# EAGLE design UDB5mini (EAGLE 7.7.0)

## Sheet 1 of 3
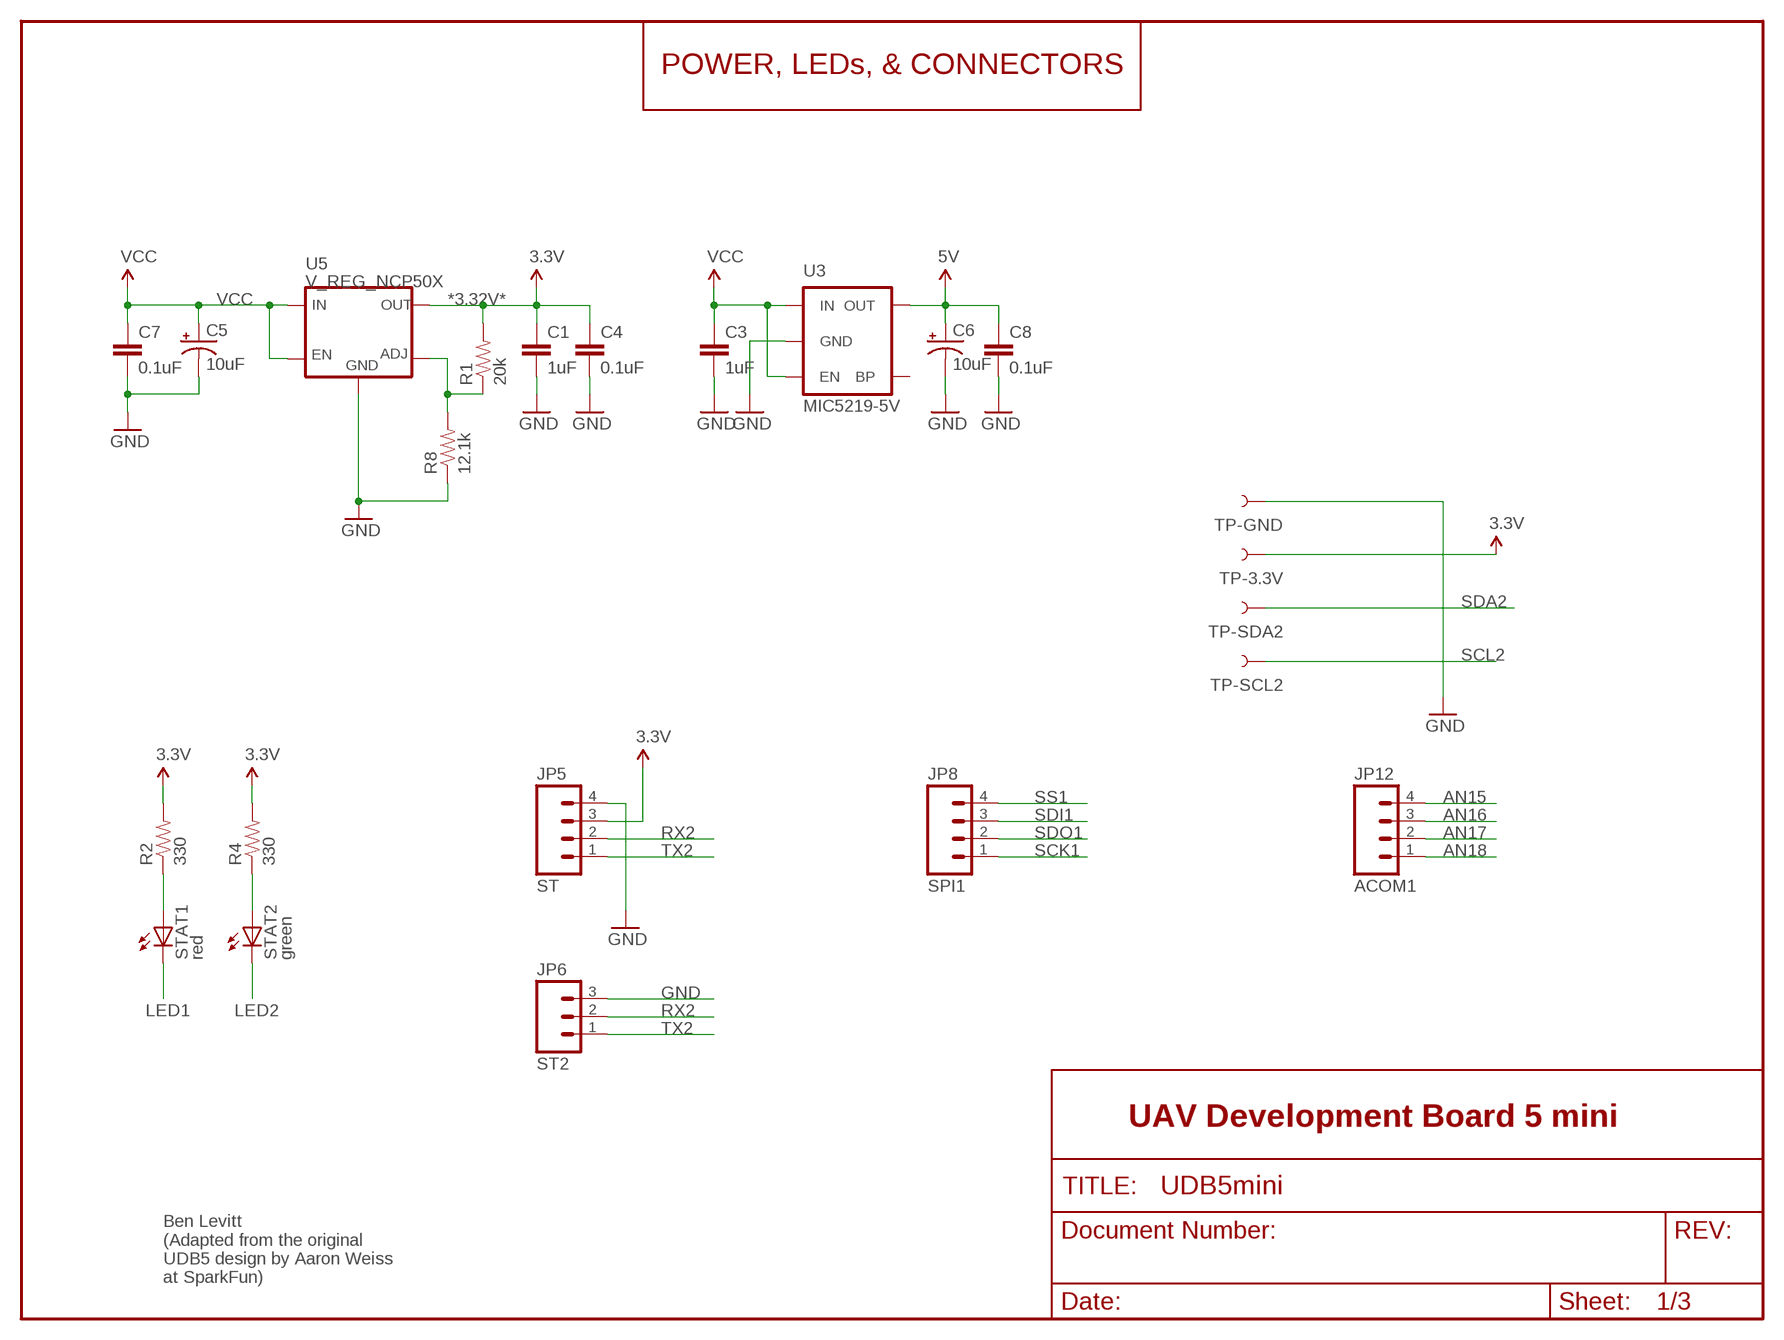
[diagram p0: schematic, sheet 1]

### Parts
C1  1uF  CAP0402-CAP  [0402-CAP]
C3  1uF  CAP0402-CAP  [0402-CAP]
C4  0.1uF  CAP0402-CAP  [0402-CAP]
C5  10uF  CAP_POL1206  [EIA3216]
C6  10uF  CAP_POL1206  [EIA3216]
C7  0.1uF  CAP0402-CAP  [0402-CAP]
C8  0.1uF  CAP0402-CAP  [0402-CAP]
JP5  ST  M04PTH  [1X04]
JP6  ST2  M03PTH  [1X03]
JP8  SPI1  M04PTH  [1X04]
JP12  ACOM1  M04PTH  [1X04]
R1  20k  RESISTOR0402-RES  [0402-RES]
R2  330  RESISTOR0402-RES  [0402-RES]
R4  330  RESISTOR0402-RES  [0402-RES]
R8  12.1k  RESISTOR0402-RES  [0402-RES]
STAT1  red  LED0603  [LED-0603]
STAT2  green  LED0603  [LED-0603]
TP-3.3V  TEST-POINT3X5  [PAD.03X.05]
TP-GND  TEST-POINT3X5  [PAD.03X.05]
TP-SCL2  TEST-POINT3X5  [PAD.03X.05]
TP-SDA2  TEST-POINT3X5  [PAD.03X.05]
U3  V_REG_LDOSMD  [SOT23-5]
U5  V_REG_NCP50X  [DPAK-5]

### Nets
3.3V: C1.1 C4.1 JP5.3 R1.2 R2.2 R4.2 TP-3.3V.P$1 U5.VOUT(OUT) ; also sheet 2,3
5V: C6.A(+) C8.1 U3.5(OUT) ; also sheet 3
AN15: JP12.4 ; also sheet 2
AN16: JP12.3 ; also sheet 2
AN17: JP12.2 ; also sheet 2
AN18: JP12.1 ; also sheet 2
GND: C1.2 C3.2 C4.2 C5.C(-) C6.C(-) C7.2 C8.2 JP5.4 JP6.3 R8.1 TP-GND.P$1 U3.2(GND) U5.GND ; also sheet 2,3
LED1: STAT1.C ; also sheet 2
LED2: STAT2.C ; also sheet 2
N$1: R2.1 STAT1.A
N$2: R4.1 STAT2.A
N$9: R1.1 R8.2 U5.ADJ
RX2: JP5.2 JP6.2 ; also sheet 2
SCK1: JP8.1 ; also sheet 2
SCL2: TP-SCL2.P$1 ; also sheet 2
SDA2: TP-SDA2.P$1 ; also sheet 2
SDI1: JP8.3 ; also sheet 2
SDO1: JP8.2 ; also sheet 2
SS1: JP8.4 ; also sheet 2
TX2: JP5.1 JP6.1 ; also sheet 2
VCC: C3.1 C5.A(+) C7.1 U3.1(IN) U3.4(EN) U5.EN U5.VIN(IN) ; also sheet 3
Unconnected: U3.3(BP)

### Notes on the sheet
- POWER, LEDs, & CONNECTORS
- *3.32V*
- MIC5219-5V
- UAV Development Board 5 mini
- Ben Levitt
  (Adapted from the original
  UDB5 design by Aaron Weiss
  at SparkFun)

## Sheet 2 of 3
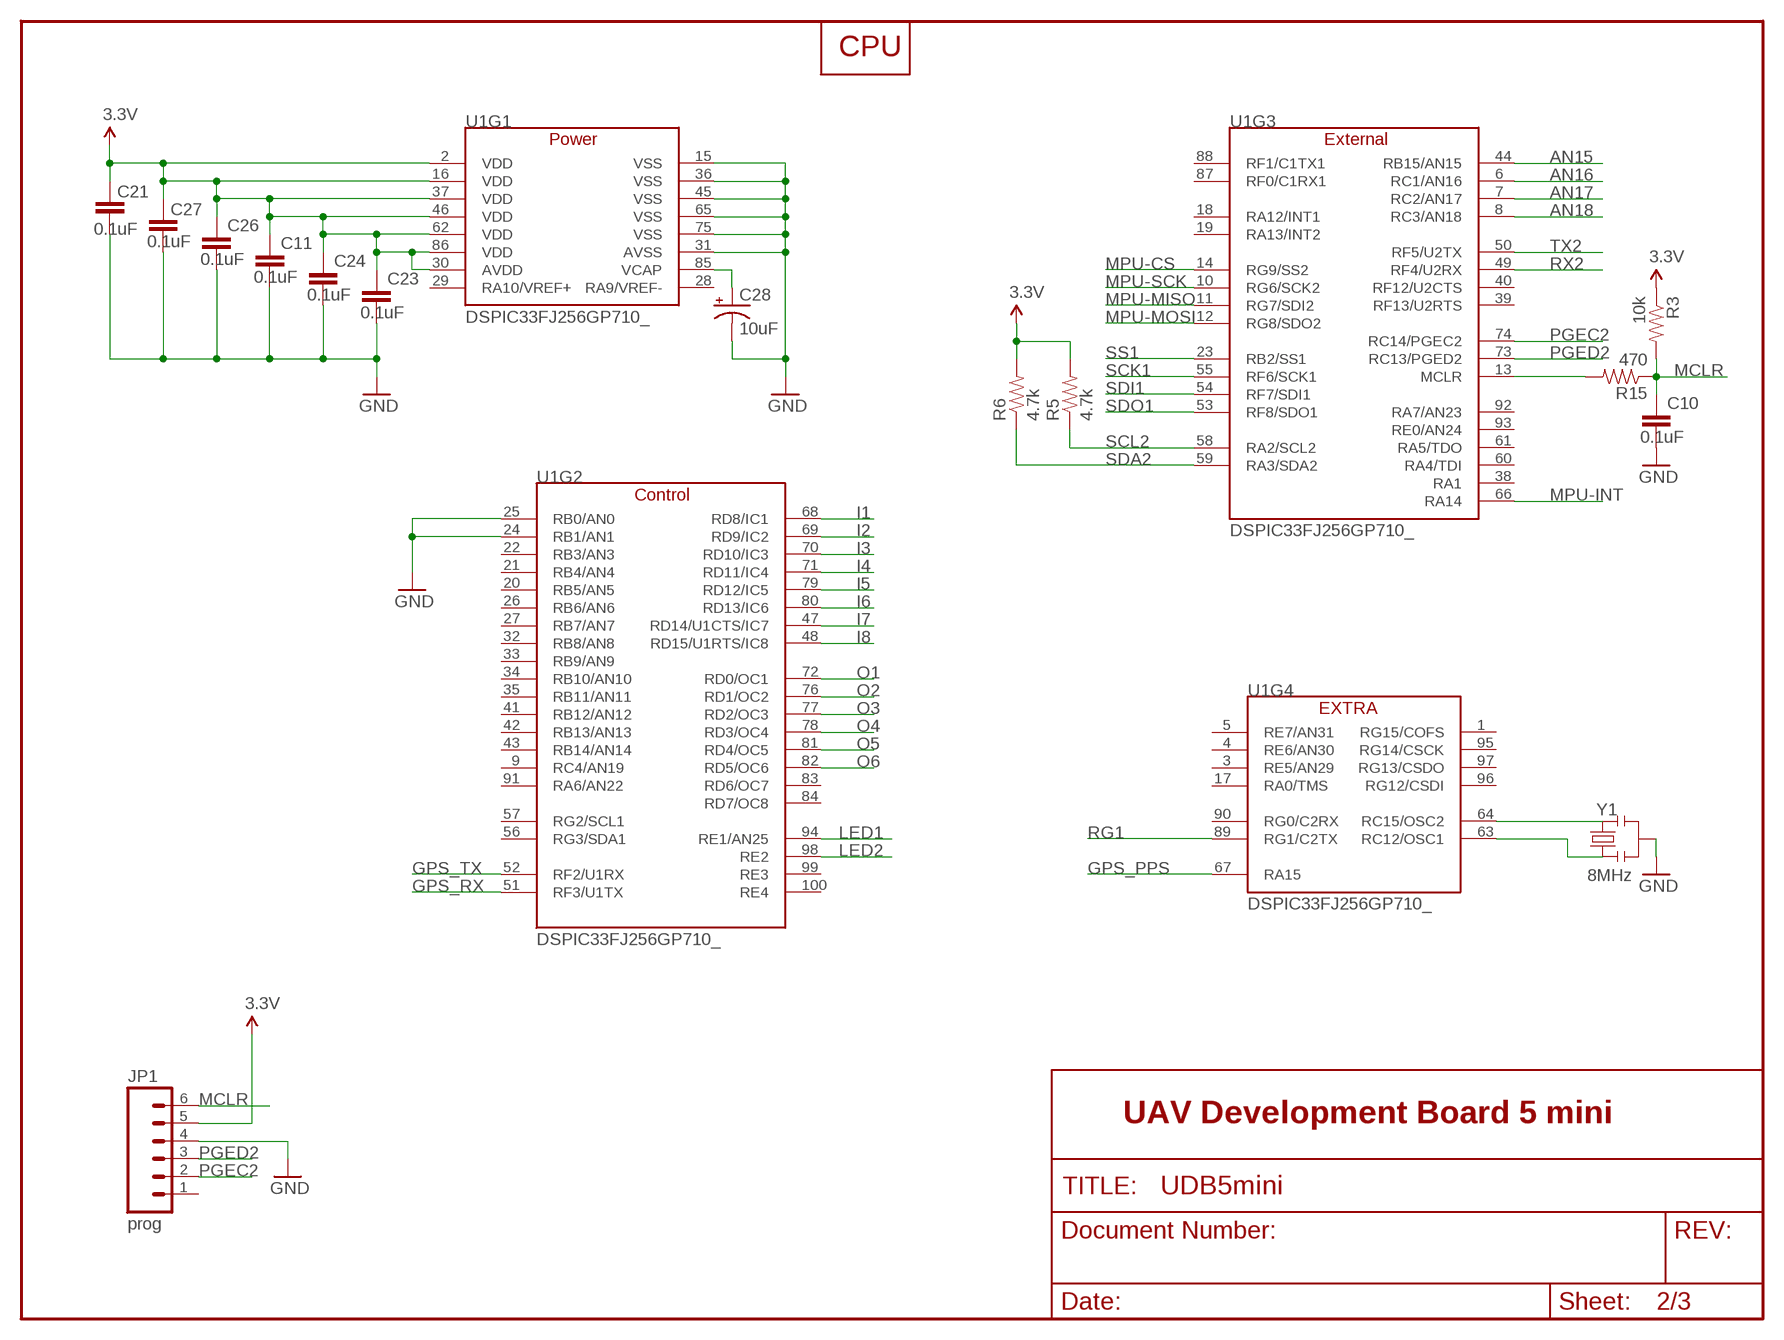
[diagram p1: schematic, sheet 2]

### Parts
C10  0.1uF  CAP0402-CAP  [0402-CAP]
C11  0.1uF  CAP0402-CAP  [0402-CAP]
C21  0.1uF  CAP0402-CAP  [0402-CAP]
C23  0.1uF  CAP0402-CAP  [0402-CAP]
C24  0.1uF  CAP0402-CAP  [0402-CAP]
C26  0.1uF  CAP0402-CAP  [0402-CAP]
C27  0.1uF  CAP0402-CAP  [0402-CAP]
C28  10uF  CAP_POL1206  [EIA3216]
JP1  prog  M06SIP  [1X06]
R3  10k  RESISTOR0402-RES  [0402-RES]
R5  4.7k  RESISTOR0402-RES  [0402-RES]
R6  4.7k  RESISTOR0402-RES  [0402-RES]
R15  470  RESISTOR0402-RES  [0402-RES]
U1  DSPIC33FJ256GP710_  [TQFP-100-12X12MM]
Y1  RESONATORSMD  [RESONATOR-SMD]

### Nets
3.3V: C11.1 C21.1 C23.1 C24.1 C26.1 C27.1 JP1.5 R3.1 R5.2 R6.2 U1.2(VDD) U1.16(VDD) U1.30(AVDD) U1.37(VDD) U1.46(VDD) U1.62(VDD) U1.86(VDD) ; also sheet 1,3
AN15: U1.44(RB15/AN15) ; also sheet 1
AN16: U1.6(RC1/AN16) ; also sheet 1
AN17: U1.7(RC2/AN17) ; also sheet 1
AN18: U1.8(RC3/AN18) ; also sheet 1
GND: C10.2 C11.2 C21.2 C23.2 C24.2 C26.2 C27.2 C28.C(-) JP1.4 U1.15(VSS) U1.24(RB1/AN1) U1.25(RB0/AN0) U1.31(AVSS) U1.36(VSS) U1.45(VSS) U1.65(VSS) U1.75(VSS) Y1.2 ; also sheet 1,3
GPS_PPS: U1.67(RA15) ; also sheet 3
GPS_RX: U1.51(RF3/U1TX) ; also sheet 3
GPS_TX: U1.52(RF2/U1RX) ; also sheet 3
I1: U1.68(RD8/IC1) ; also sheet 3
I2: U1.69(RD9/IC2) ; also sheet 3
I3: U1.70(RD10/IC3) ; also sheet 3
I4: U1.71(RD11/IC4) ; also sheet 3
I5: U1.79(RD12/IC5) ; also sheet 3
I6: U1.80(RD13/IC6) ; also sheet 3
I7: U1.47(RD14/U1CTS/IC7) ; also sheet 3
I8: U1.48(RD15/U1RTS/IC8) ; also sheet 3
LED1: U1.94(RE1/AN25) ; also sheet 1
LED2: U1.98(RE2) ; also sheet 1
MCLR: C10.1 JP1.6 R3.2 R15.1
MPU-CS: U1.14(RG9/SS2) ; also sheet 3
MPU-INT: U1.66(RA14) ; also sheet 3
MPU-MISO: U1.11(RG7/SDI2) ; also sheet 3
MPU-MOSI: U1.12(RG8/SDO2) ; also sheet 3
MPU-SCK: U1.10(RG6/SCK2) ; also sheet 3
N$3: U1.64(RC15/OSC2) Y1.3
N$6: U1.63(RC12/OSC1) Y1.1
N$7: R15.2 U1.13(MCLR)
N$35: C28.A(+) U1.85(VCAP)
O1: U1.72(RD0/OC1) ; also sheet 3
O2: U1.76(RD1/OC2) ; also sheet 3
O3: U1.77(RD2/OC3) ; also sheet 3
O4: U1.78(RD3/OC4) ; also sheet 3
O5: U1.81(RD4/OC5) ; also sheet 3
O6: U1.82(RD5/OC6) ; also sheet 3
PGEC2: JP1.2 U1.74(RC14/PGEC2)
PGED2: JP1.3 U1.73(RC13/PGED2)
RG1: U1.89(RG1/C2TX) ; also sheet 3
RX2: U1.49(RF4/U2RX) ; also sheet 1
SCK1: U1.55(RF6/SCK1) ; also sheet 1
SCL2: R5.1 U1.58(RA2/SCL2) ; also sheet 1
SDA2: R6.1 U1.59(RA3/SDA2) ; also sheet 1
SDI1: U1.54(RF7/SDI1) ; also sheet 1
SDO1: U1.53(RF8/SDO1) ; also sheet 1
SS1: U1.23(RB2/SS1) ; also sheet 1
TX2: U1.50(RF5/U2TX) ; also sheet 1
Unconnected: JP1.1 U1.1(RG15/COFS) U1.3(RE5/AN29) U1.4(RE6/AN30) U1.5(RE7/AN31) U1.9(RC4/AN19) U1.17(RA0/TMS) U1.18(RA12/INT1) U1.19(RA13/INT2) U1.20(RB5/AN5) U1.21(RB4/AN4) U1.22(RB3/AN3) U1.26(RB6/AN6) U1.27(RB7/AN7) U1.28(RA9/VREF-) U1.29(RA10/VREF+) U1.32(RB8/AN8) U1.33(RB9/AN9) U1.34(RB10/AN10) U1.35(RB11/AN11) U1.38(RA1) U1.39(RF13/U2RTS) U1.40(RF12/U2CTS) U1.41(RB12/AN12) U1.42(RB13/AN13) U1.43(RB14/AN14) U1.56(RG3/SDA1) U1.57(RG2/SCL1) U1.60(RA4/TDI) U1.61(RA5/TDO) U1.83(RD6/OC7) U1.84(RD7/OC8) U1.87(RF0/C1RX1) U1.88(RF1/C1TX1) U1.90(RG0/C2RX) U1.91(RA6/AN22) U1.92(RA7/AN23) U1.93(RE0/AN24) U1.95(RG14/CSCK) U1.96(RG12/CSDI) U1.97(RG13/CSDO) U1.99(RE3) U1.100(RE4)

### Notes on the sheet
- CPU
- 8MHz
- UAV Development Board 5 mini

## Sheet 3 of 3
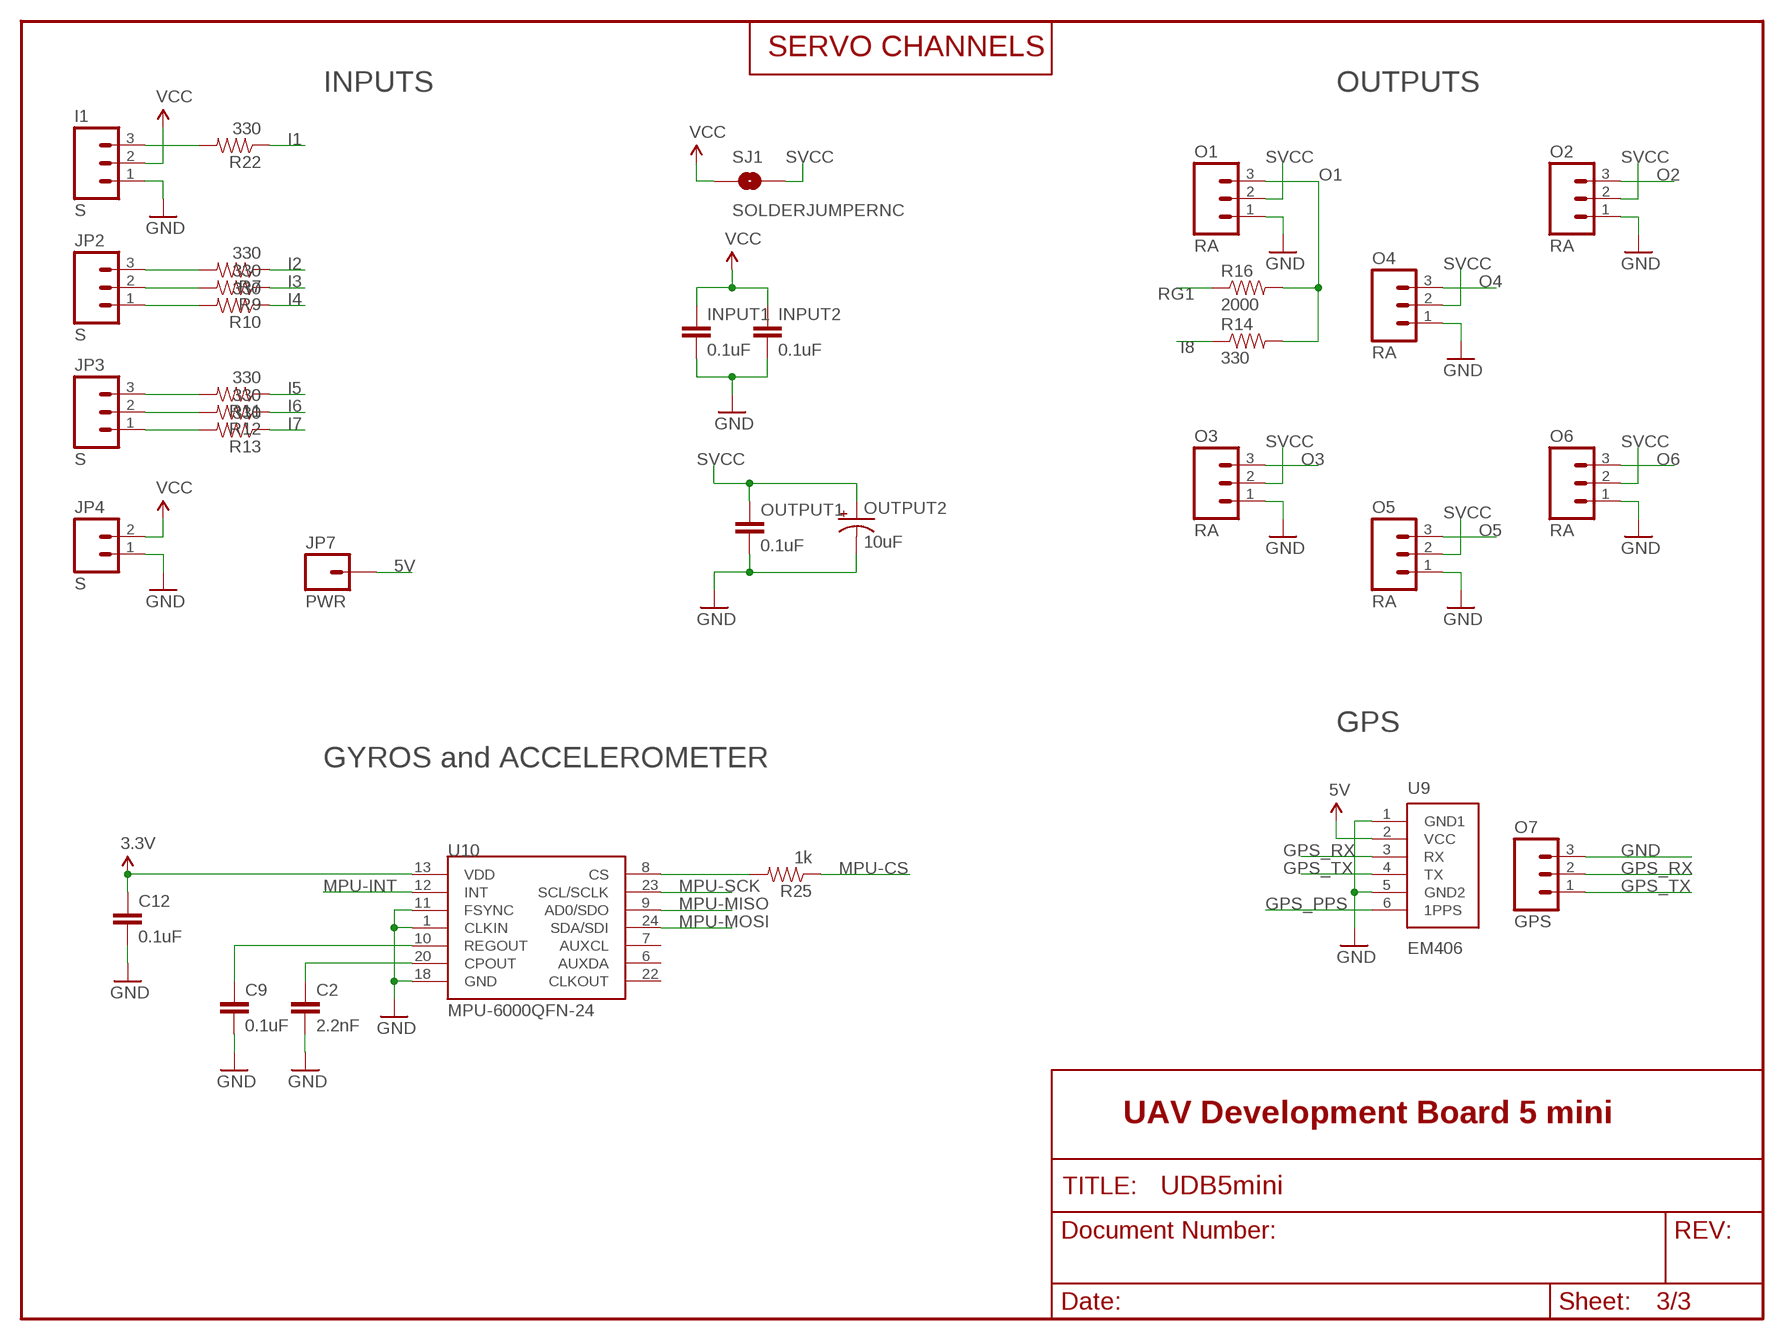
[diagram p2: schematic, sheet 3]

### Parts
C2  2.2nF  CAP0402-CAP  [0402-CAP]
C9  0.1uF  CAP0402-CAP  [0402-CAP]
C12  0.1uF  CAP0402-CAP  [0402-CAP]
I1  S  M03PTH  [1X03]
INPUT1  0.1uF  CAP0402-CAP  [0402-CAP]
INPUT2  0.1uF  CAP0402-CAP  [0402-CAP]
JP2  S  M03PTH  [1X03]
JP3  S  M03PTH  [1X03]
JP4  S  M02PTH  [1X02]
JP7  PWR  M01PTH  [1X01]
O1  RA  M03PTH  [1X03]
O2  RA  M03PTH  [1X03]
O3  RA  M03PTH  [1X03]
O4  RA  M03PTH  [1X03]
O5  RA  M03PTH  [1X03]
O6  RA  M03PTH  [1X03]
O7  GPS  M03PTH  [1X03]
OUTPUT1  0.1uF  CAP0402-CAP  [0402-CAP]
OUTPUT2  10uF  CAP_POL1206  [EIA3216]
R7  330  RESISTOR0402-RES  [0402-RES]
R9  330  RESISTOR0402-RES  [0402-RES]
R10  330  RESISTOR0402-RES  [0402-RES]
R11  330  RESISTOR0402-RES  [0402-RES]
R12  330  RESISTOR0402-RES  [0402-RES]
R13  330  RESISTOR0402-RES  [0402-RES]
R14  330  RESISTOR0402-RES  [0402-RES]
R16  2000  RESISTOR0402-RES  [0402-RES]
R22  330  RESISTOR0402-RES  [0402-RES]
R25  1k  RESISTOR0402-RES  [0402-RES]
SJ1  SOLDERJUMPERNC  [SJ_2S]
U9  EM406  [EM406]
U10  MPU-6000QFN-24  [QFN-24-TESTING]

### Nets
3.3V: C12.1 U10.13(VDD) ; also sheet 1,2
5V: JP7.1 U9.2(VCC) ; also sheet 1
GND: C2.2 C9.2 C12.2 I1.1 INPUT1.2 INPUT2.2 JP4.1 O1.1 O2.1 O3.1 O4.1 O5.1 O6.1 O7.3 OUTPUT1.2 OUTPUT2.C(-) U9.1(GND1) U9.5(GND2) U10.1(CLKIN) U10.11(FSYNC) U10.18(GND) ; also sheet 1,2
GPS_PPS: U9.6(1PPS) ; also sheet 2
GPS_RX: O7.2 U9.3(RX) ; also sheet 2
GPS_TX: O7.1 U9.4(TX) ; also sheet 2
I1: R22.1 ; also sheet 2
I2: R7.1 ; also sheet 2
I3: R9.1 ; also sheet 2
I4: R10.1 ; also sheet 2
I5: R11.1 ; also sheet 2
I6: R12.1 ; also sheet 2
I7: R13.1 ; also sheet 2
I8: R14.1 ; also sheet 2
MPU-CS: R25.1 ; also sheet 2
MPU-INT: U10.12(INT) ; also sheet 2
MPU-MISO: U10.9(AD0/SDO) ; also sheet 2
MPU-MOSI: U10.24(SDA/SDI) ; also sheet 2
MPU-SCK: U10.23(SCL/SCLK) ; also sheet 2
N$4: JP2.3 R7.2
N$5: R25.2 U10.8(CS)
N$8: JP2.2 R9.2
N$10: JP2.1 R10.2
N$11: JP3.3 R11.2
N$12: JP3.2 R12.2
N$13: C2.1 U10.20(CPOUT)
N$14: JP3.1 R13.2
N$16: C9.1 U10.10(REGOUT)
N$21: I1.3 R22.2
O1: O1.3 R14.2 R16.2 ; also sheet 2
O2: O2.3 ; also sheet 2
O3: O3.3 ; also sheet 2
O4: O4.3 ; also sheet 2
O5: O5.3 ; also sheet 2
O6: O6.3 ; also sheet 2
RG1: R16.1 ; also sheet 2
SVCC: O1.2 O2.2 O3.2 O4.2 O5.2 O6.2 OUTPUT1.1 OUTPUT2.A(+) SJ1.2
VCC: I1.2 INPUT1.1 INPUT2.1 JP4.2 SJ1.1 ; also sheet 1
Unconnected: U10.6(AUXDA) U10.7(AUXCL) U10.22(CLKOUT)

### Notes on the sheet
- SERVO CHANNELS
- INPUTS | OUTPUTS
- GPS
- GYROS and ACCELEROMETER
- UAV Development Board 5 mini

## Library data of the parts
C1 C3 C4 C7 C8 C10 C11 C21 C23 C24 C26 C27 INPUT1 INPUT2 OUTPUT1 = SparkFun:CAP: Capacitor
C2 C9 C12 = SparkFun-Capacitors:CAP: Capacitor
C5 C6 C28 OUTPUT2 = SparkFun:CAP_POL: Capacitor Polarized
I1 JP2 JP3 O1-O7 = SparkFun:M03: Header 3 Standard 3-pin 0.1" header. Use with straight break away headers (SKU : PRT-00116), right angle break away headers (PRT-00553), swiss pins (PRT-00743), machine pins (PRT-00117), and female headers (PRT-00115). Molex polarized connector foot print use with SKU : PRT-08232 with associated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
JP1 = SparkFun:M06: Header 6 Standard 6-pin 0.1" header. Use with straight break away headers (SKU : PRT-00116), right angle break away headers (PRT-00553), swiss pins (PRT-00743), machine pins (PRT-00117), and female headers (PRT-00115). Molex polarized connector foot print use with SKU : PRT-08094 with associated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
JP4 = SparkFun-Connectors:M02: Standard 2-pin 0.1" header. Use with
JP5 JP8 JP12 = udb5mini:M04: Header 4 Standard 4-pin 0.1" header. Use with straight break away headers (SKU : PRT-00116), right angle break away headers (PRT-00553), swiss pins (PRT-00743), machine pins (PRT-00117), and female headers (PRT-00115). Molex polarized connector foot print use with SKU : PRT-08231 with associated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
JP6 = SparkFun-Connectors:M03: Header 3 Standard 3-pin 0.1" header. Use with straight break away headers (SKU : PRT-00116), right angle break away headers (PRT-00553), swiss pins (PRT-00743), machine pins (PRT-00117), and female headers (PRT-00115). Molex polarized connector foot print use with SKU : PRT-08232 with associated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
JP7 = SparkFun-Connectors:M01: Header 1
R1-R16 R22 R25 = SparkFun:RESISTOR: Resistor
SJ1 = SparkFun:SOLDERJUMPER: Solder Jumper
STAT1 STAT2 = SparkFun:LED: LEDs
TP-3.3V TP-GND TP-SCL2 TP-SDA2 = SparkFun-Passives:TEST-POINT: Bare copper test points for troubleshooting or ICT
U1 = SparkFun:DSPIC33FJ256GP710
U3 = SparkFun-PowerIC:V_REG_LDO: Voltage Regulator LDO Standard 150mA LDO voltage regulator in SOT-23 layout. Micrel part MIC5205. BP (by-pass) pin is used to lower output noise with 470pF cap.
U5 = SparkFun:V_REG_NCP50X: NCP550x 500mA LDO Voltage Regulator
U9 = SparkFun:EM406: EM406 Connector Proven layout and schematic for EM406 connector. Spark Fun Electronics SKU : GPS-00579
U10 = SparkFun-Sensors:MPU-6000: MPU-6000 - I2C address is 0x68 with AD0 low and 0x69 with AD0 high.
Y1 = SparkFun:RESONATOR: Resonator Small SMD resonator. This is the itty bitty 10/20MHz resonators with built in caps. CSTCE10M0G55 and CSTCE20M0V53. Footprint has been reviewed closely but hasn't been tested yet.

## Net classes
1 antenna: width 2.974 mm

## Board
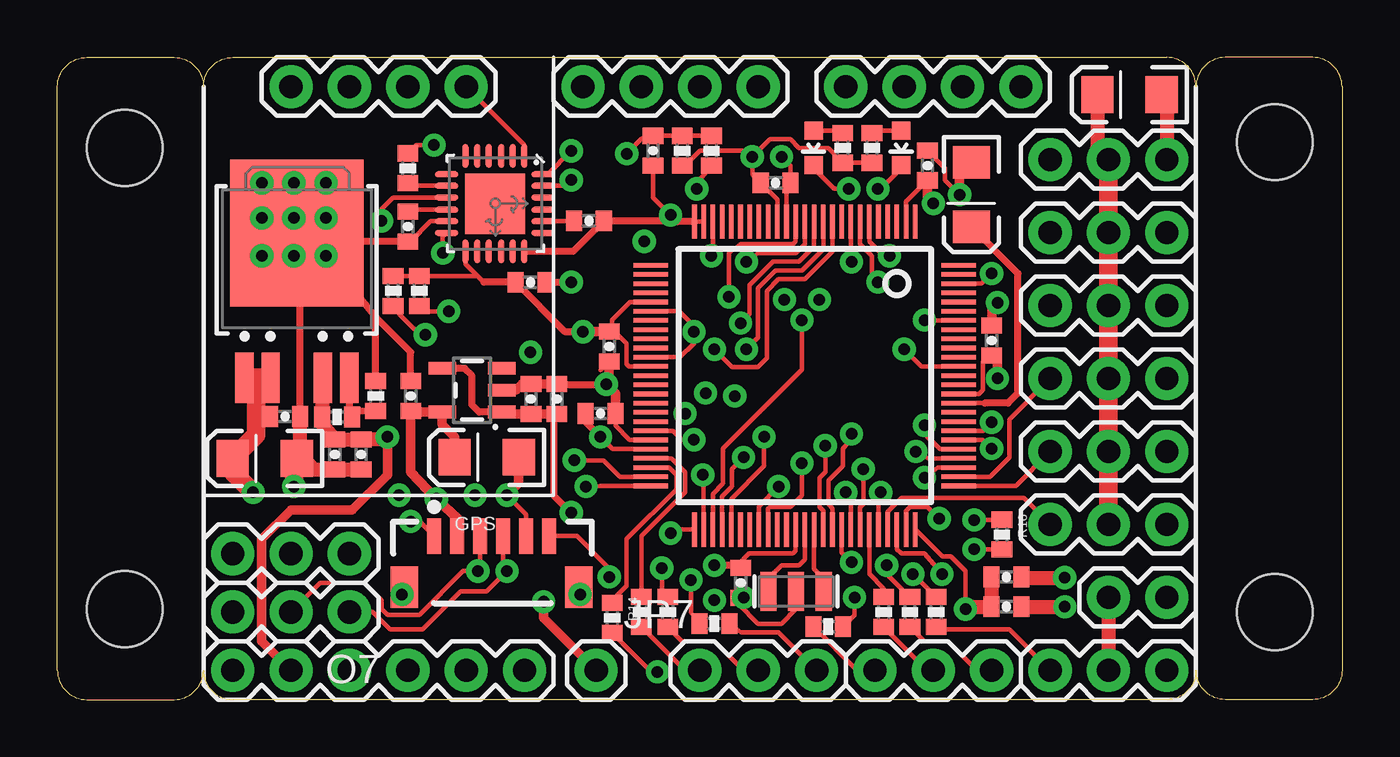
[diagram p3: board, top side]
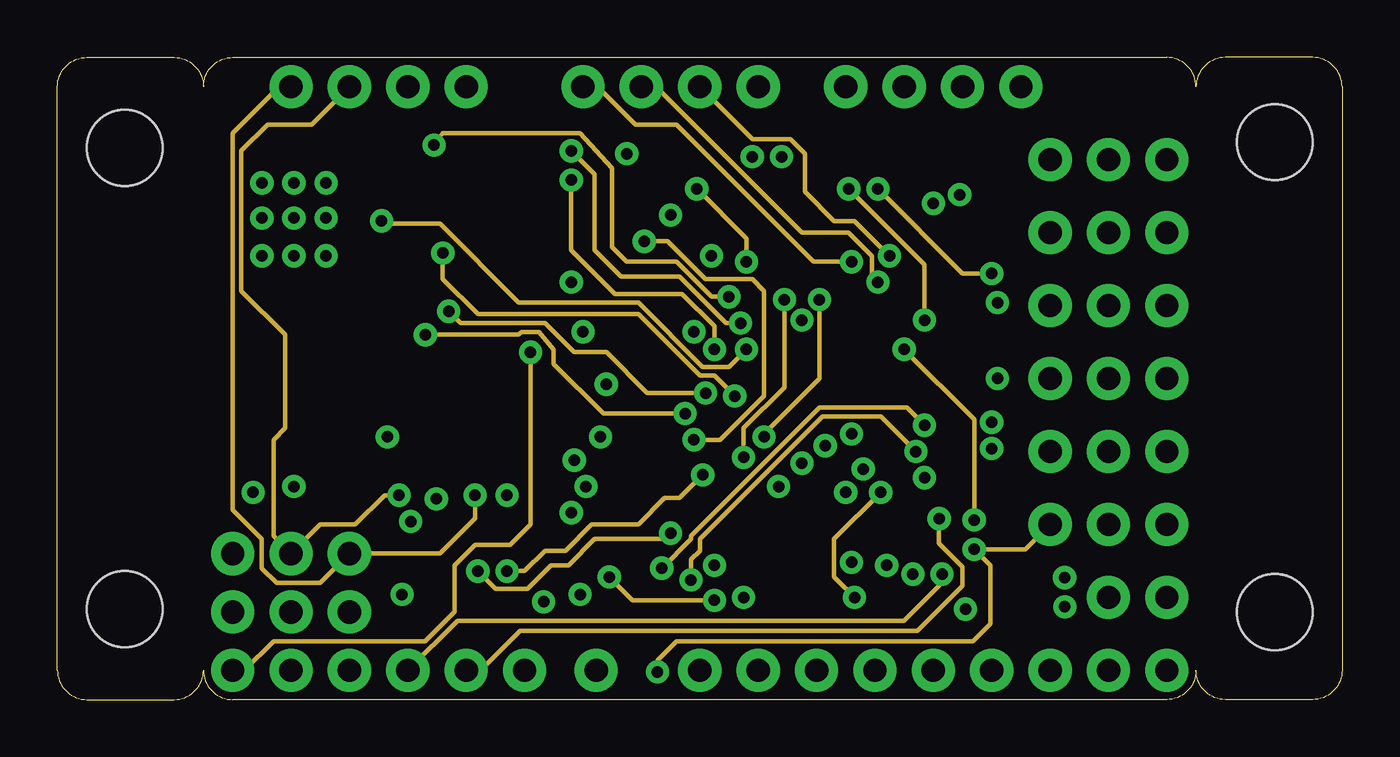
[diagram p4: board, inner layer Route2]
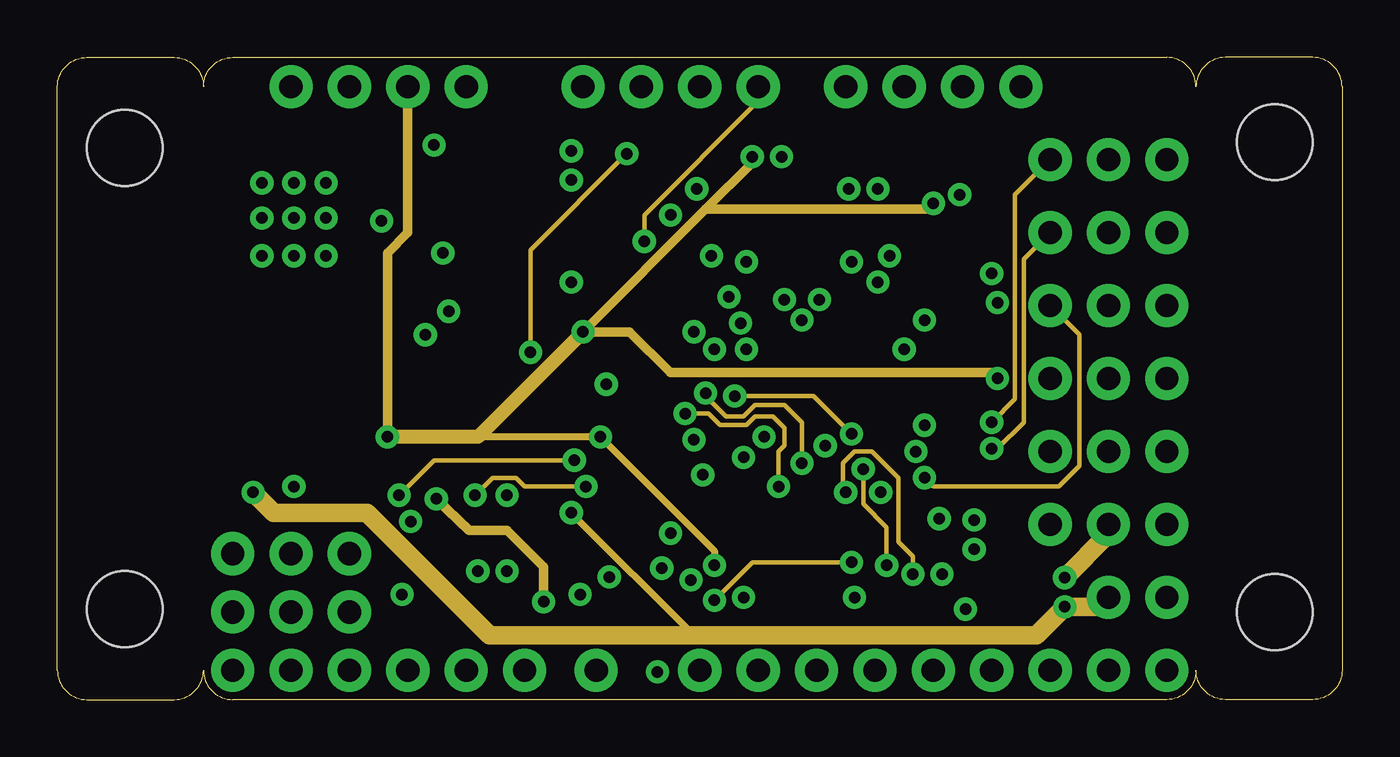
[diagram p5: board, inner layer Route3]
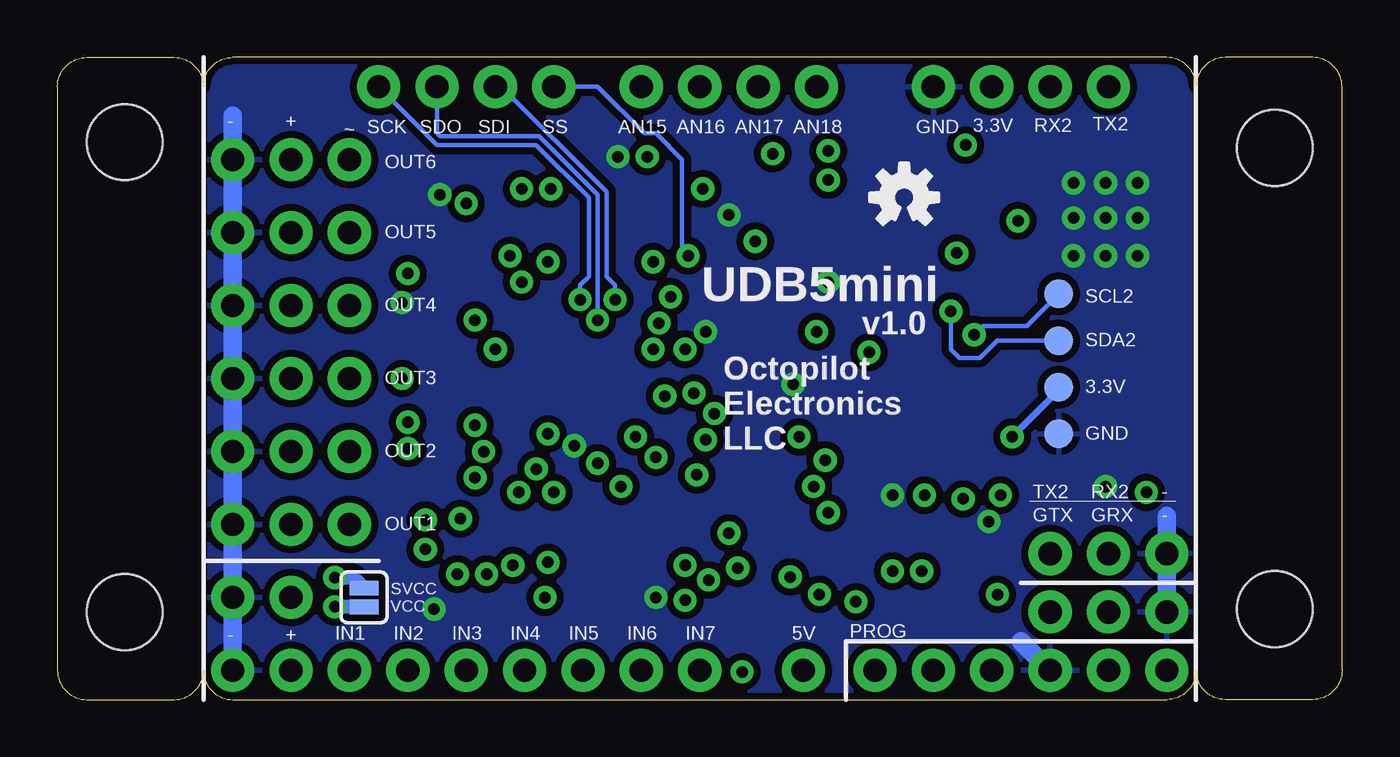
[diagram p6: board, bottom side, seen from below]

Size 55.88 x 27.94 mm. Coordinates in mm from the lower left corner, seen from the top.
Outline: 0,1.27 0,26.67 arc-90 1.27,27.94 5.08,27.94 arc-90 6.35,26.67 arc-90 7.62,27.94 48.26,27.94 arc-90 49.53,26.67 arc-90 50.8,27.94 54.61,27.94 arc-90 55.88,26.67 55.88,1.27 arc-90 54.61,0 50.8,0 arc-90 49.53,1.27 arc-90 48.26,0 7.62,0 arc-90 6.35,1.27 arc-90 5.08,0 1.27,0 arc-90 0,1.27
Copper layers (1*2*3*16): Top 0.035mm / dielectric 0.23mm / Route2 0.035mm / dielectric 0.93mm / Route3 0.035mm / dielectric 0.23mm / Bottom 0.035mm
Design rules "BatchPCB-4-layer *": minimum track width 5mil, minimum drill 12mil, track to track 5mil, track to pad 5mil, pad to pad 5mil, via to via 5mil, smd to smd 5mil, copper to edge 8mil, drill to drill 12mil, minimum pad ring 12mil, minimum via ring 10mil, stop-mask expansion 4mil, vias tented up to drill 20mil, thermal gap 12mil

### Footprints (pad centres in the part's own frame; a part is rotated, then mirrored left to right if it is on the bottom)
0402-CAP = smd 0.7 x 0.9: 1 -0.65,0; 2 0.65,0
EIA3216 = smd 1.4 x 1.6: A 1.4,0; C -1.4,0
1X03 = drill 1.016 pad 1.88: 1 0,0; 2 2.54,0; 3 5.08,0
1X06 = drill 1.016 pad 1.88: 1 0,0; 2 2.54,0; 3 5.08,0; 4 7.62,0; 5 10.16,0; 6 12.7,0
1X02 = drill 1.016 pad 1.88: 1 0,0; 2 2.54,0
1X04 = drill 1.016 pad 1.88: 1 0,0; 2 2.54,0; 3 5.08,0; 4 7.62,0
1X01 = drill 1.016 pad 1.88: 1 0,0
0402-RES = smd 0.7 x 0.9: 1 -0.65,0; 2 0.65,0
SJ_2S = smd 0.635 x 1.27: 1 -0.412,0; 2 0.412,0
LED-0603 = smd 0.8 x 0.8: A 0,-0.75; C 0,0.75
PAD.03X.05 = smd 1.27 x 1.27: P$1 0,0
TQFP-100-12X12MM = smd 1.5 x 0.2: 1 -6.7,4.8; 2 -6.7,4.4; 3 -6.7,4; 4 -6.7,3.6; 5 -6.7,3.2; 6 -6.7,2.8; 7 -6.7,2.4; 8 -6.7,2; 9 -6.7,1.6; 10 -6.7,1.2; 11 -6.7,0.8; 12 -6.7,0.4; 13 -6.7,0; 14 -6.7,-0.4; 15 -6.7,-0.8; 16 -6.7,-1.2; 17 -6.7,-1.6; 18 -6.7,-2; 19 -6.7,-2.4; 20 -6.7,-2.8; 21 -6.7,-3.2; 22 -6.7,-3.6; 23 -6.7,-4; 24 -6.7,-4.4; 25 -6.7,-4.8; 51 6.7,-4.8; 52 6.7,-4.4; 53 6.7,-4; 54 6.7,-3.6; 55 6.7,-3.2; 56 6.7,-2.8; 57 6.7,-2.4; 58 6.7,-2; 59 6.7,-1.6; 60 6.7,-1.2; 61 6.7,-0.8; 62 6.7,-0.4; 63 6.7,0; 64 6.7,0.4; 65 6.7,0.8; 66 6.7,1.2; 67 6.7,1.6; 68 6.7,2; 69 6.7,2.4; 70 6.7,2.8; 71 6.7,3.2; 72 6.7,3.6; 73 6.7,4; 74 6.7,4.4; 75 6.7,4.8 | smd 0.2 x 1.5: 26 -4.8,-6.7; 27 -4.4,-6.7; 28 -4,-6.7; 29 -3.6,-6.7; 30 -3.2,-6.7; 31 -2.8,-6.7; 32 -2.4,-6.7; 33 -2,-6.7; 34 -1.6,-6.7; 35 -1.2,-6.7; 36 -0.8,-6.7; 37 -0.4,-6.7; 38 0,-6.7; 39 0.4,-6.7; 40 0.8,-6.7; 41 1.2,-6.7; 42 1.6,-6.7; 43 2,-6.7; 44 2.4,-6.7; 45 2.8,-6.7; 46 3.2,-6.7; 47 3.6,-6.7; 48 4,-6.7; 49 4.4,-6.7; 50 4.8,-6.7; 76 4.8,6.7; 77 4.4,6.7; 78 4,6.7; 79 3.6,6.7; 80 3.2,6.7; 81 2.8,6.7; 82 2.4,6.7; 83 2,6.7; 84 1.6,6.7; 85 1.2,6.7; 86 0.8,6.7; 87 0.4,6.7; 88 0,6.7; 89 -0.4,6.7; 90 -0.8,6.7; 91 -1.2,6.7; 92 -1.6,6.7; 93 -2,6.7; 94 -2.4,6.7; 95 -2.8,6.7; 96 -3.2,6.7; 97 -3.6,6.7; 98 -4,6.7; 99 -4.4,6.7; 100 -4.8,6.7
SOT23-5 = smd 0.55 x 1.2: 1 -0.95,-1.3; 2 0,-1.3; 3 0.95,-1.3; 4 0.95,1.3; 5 -0.95,1.3
DPAK-5 = smd 0.8 x 2.2: ADJ 2.28,-5.3; EN -2.28,-5.3; VIN -1.14,-5.3; VOUT 1.14,-5.3 | smd 5.8 x 6.4: GND 0,1
EM406 = smd 0.6 x 1.55: 1 0,0; 2 1,0; 3 2,0; 4 3,0; 5 4,0; 6 5,0 | smd 1.2 x 1.8: P$1 -1.3,-2.225; P$2 6.3,-2.225
QFN-24-TESTING = smd 1.016 x 0.254: 1 -2.066,1.257; 2 -2.066,0.75; 3 -2.066,0.247; 4 -2.066,-0.287; 5 -2.066,-0.792; 6 -2.066,-1.297; 13 2.086,-1.297; 14 2.086,-0.792; 15 2.086,-0.287; 16 2.086,0.247; 17 2.086,0.75; 18 2.086,1.257 | smd 0.254 x 1.016: 7 -1.267,-2.122; 8 -0.762,-2.122; 9 -0.258,-2.122; 10 0.278,-2.122; 11 0.78,-2.122; 12 1.287,-2.122; 19 1.287,2.082; 20 0.78,2.082; 21 0.278,2.082; 22 -0.258,2.082; 23 -0.762,2.082; 24 -1.267,2.082 | smd 2.616 x 2.616: P$1 0.02,-0.01
STAND-OFF = hole 3.302: 0,0
RESONATOR-SMD = smd 0.7 x 1.7: 1 -1.2,0; 2 0,0; 3 1.2,0

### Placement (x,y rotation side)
C1  12.06,10.67 270 top
C2  23.11,20.83 0 top
C3  21.72,13.08 90 top
C4  13.21,10.67 270 top
C5  9.02,10.49 180 top
C6  18.67,10.54 180 top
C7  9.91,12.32 0 top
C8  15.37,13.21 90 top
C9  15.24,20.57 270 top
C10  25.91,23.88 270 top
C11  23.62,12.45 0 top
C12  20.57,18.16 0 top
C21  37.85,23.24 90 top
C23  40.64,15.62 90 top
C24  29.72,5.08 270 top
C26  24,15.37 270 top
C27  31.24,22.48 0 top
C28  39.75,21.97 270 top
I1  48.26,1.27 180 top
INPUT1  41.27,4.04 180 top
INPUT2  20.6,13.08 90 top
JP1  20.32,1.27 180 top
JP2  35.56,1.27 0 top
JP3  27.94,1.27 0 top
JP4  48.26,4.45 180 top
JP5  10.16,26.67 0 top
JP6  12.7,6.35 180 top
JP7  23.43,1.27 0 top
JP8  41.91,26.67 180 top
JP12  22.86,26.67 0 top
O1  48.26,7.62 180 top
O2  48.26,10.79 180 top
O3  48.26,13.97 180 top
O4  48.26,17.14 180 top
O5  48.26,20.32 180 top
O6  48.26,23.5 180 top
O7  12.7,3.81 180 top
OUTPUT1  41.27,5.33 180 top
OUTPUT2  46.63,26.31 180 top
R1  12.17,12.29 180 top
R2  34.16,24 270 top
R3  27.18,23.88 90 top
R4  35.43,24 270 top
R5  14.61,17.78 90 top
R6  15.75,17.78 90 top
R7  37.08,3.81 270 top
R8  13.84,13.21 270 top
R9  35.94,3.81 270 top
R10  33.53,3.17 180 top
R11  28.57,3.3 0 top
R12  26.54,3.81 270 top
R13  25.4,3.81 270 top
R14  24.13,3.56 270 top
R15  28.45,23.88 270 top
R16  41.08,7.18 270 top
R22  38.23,3.81 270 top
R25  15.24,23.11 270 top
SJ1  42.55,4.45 90 bottom
STAT1  32.89,24 180 top
STAT2  36.7,24 180 top
TP-3.3V  12.32,13.59 0 bottom
TP-GND  12.32,11.56 0 bottom
TP-SCL2  12.32,17.65 0 bottom
TP-SDA2  12.32,15.62 0 bottom
U1  32.51,14.1 270 top
U3  18.03,13.46 90 top
U5  10.41,19.3 0 top
U9  16.38,7.11 0 top
U10  19.05,21.59 270 top
U$2  [OSHW-LOGO-S]  19.05,21.84 0 bottom
U$3  [STAND-OFF]  2.92,24 0 top
U$4  [STAND-OFF]  2.92,3.94 0 top
U$5  [STAND-OFF]  52.96,3.81 0 top
U$6  [STAND-OFF]  52.96,24.26 0 top
Y1  32.13,4.7 0 top

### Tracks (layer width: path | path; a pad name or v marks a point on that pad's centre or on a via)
3.3V  (via drill 0.5)
  Top 0.203: U1.62 32.11,6.46 32,6.35 30.08,6.35 29.58,5.84 29.21,5.84 | U1.30 24.92,17.3 24.13,16.51 24.13,16.14 C26.1 24.24,16.02 24.77,15.49 24.77,14.61 24.87,14.5 U1.37 | 30.08,23.48 v30.23,23.62 | U1.2 36.91,21.67 37.7,22.46 C21.1 37.59,22.46 | v30.23,23.62 30.99,24.38 31.88,24.38 32.26,24 33.53,24 34.16,23.37 R2.2 R4.2 | v23.62,11.43 24.16,10.9 U1.46 | U1.86 40.09,13.3 40.26,13.46 40.26,14.72 C23.1 | v30.23,23.62 29.97,23.88 27.94,23.88 27.18,23.11 R3.1 | U1.16 31.31,21.76 C27.1 30.23,22.84 v30.23,23.62 | U10.13 17.75,18.95 18.27,18.43 | R5.2 R6.2 18.27,18.43 | 18.54,18.16 18.27,18.43
  Top 0.305: U5.VOUT 11.52,13.97 | v23.62,11.43 22.97,12.08 C11.1 | C24.1 29.35,5.84 29.21,5.84 v28.57,5.84 | 40.89,14.59 40.64,14.84 C23.1 | v22.86,16 22.08,16 C12.1 18.54,18.16
  Top 0.406: JP1.5 8.89,2.54 8.89,6.99 10.16,8.26 12.83,8.26 14.35,9.78 v14.35,11.43 | v40.89,13.97 40.89,14.59 | v38.1,21.59 37.85,21.84 C21.1 | 22.97,15.89 23.1,16.02 C26.1
  Top 0.61: v14.35,11.43 14.11,11.32 C4.1 C1.1 11.52,11.99 R1.2 11.52,13.97 | v22.86,16 22.97,15.89
  Route3 0.305: 18.03,11.43 v23.62,11.43 28.57,6.48 v28.57,5.84
  Route3 0.406: v30.23,23.62 30.23,23.37 28.19,21.34 | 28.19,21.34 v22.86,16 24.89,16 26.67,14.22 40.64,14.22 v40.89,13.97 | v38.1,21.59 37.85,21.34 28.19,21.34 | v14.35,11.43 14.35,19.43 15.24,20.32 JP5.3
  Route3 0.61: v22.86,16 18.29,11.43 18.03,11.43 v14.35,11.43
  Bottom 0.305: v14.35,11.43 12.32,13.46 TP-3.3V.P$1
5V  (via drill 0.5)
  Top 0.203: C6.A 16.89,10.92
  Top 0.406: U9.2 17.4,7.51 17.4,7.87 16.57,8.64 v16.48,8.73 15.37,9.91 C8.1 15.41,12.51 U3.5 16.73,11.97 17.27,11.43 17.27,11.31 16.89,10.92 | JP7.1 21.14,3.56 v21.14,4.25
  Route3 0.406: v21.14,4.25 21.14,5.78 19.56,7.37 17.91,7.37 v16.48,8.73
AN15  (via drill 0.5)
  Top 0.203: U1.44 26.78,11.7 27.18,11.3 v27.69,11.3
  Route2 0.203: v25.53,19.94 26.54,19.94 28.19,18.29 30.23,18.29 30.73,17.78 30.73,13.21 28.83,11.3 v27.69,11.3
  Route3 0.203: JP12.4 30.48,26.04 25.53,21.08 v25.53,19.94
AN16  (via drill 0.5)
  Top 0.203: U1.6 35.31,19.93 35.81,19.43 v36.2,19.3
  Route2 0.203: v36.2,19.3 34.67,20.83 33.78,20.83 32.51,22.1 32.51,23.75 31.88,24.38 30.23,24.38 JP12.3
AN17  (via drill 0.5)
  Top 0.203: U1.7 34.91,19.82 35.43,19.3 35.43,18.41 v35.69,18.16
  Route2 0.203: JP12.2 26.04,26.67 32.38,20.32 34.42,20.32 35.43,19.3 35.43,18.41 v35.69,18.16
AN18  (via drill 0.5)
  Top 0.203: U1.8 34.51,19.21 v34.54,19.05
  Route2 0.203: JP12.1 23.5,26.67 25.15,25.02 26.92,25.02 32.89,19.05 v34.54,19.05
GND  (via drill 0.5)
  Top 0.203: U1.36 27.09,14.9 27.69,15.49 v27.69,16 27.69,16.26 27.05,16.9 U1.31 | C26.2 23.62,14.34 | Y1.2 32.13,3.94 31.5,3.3 30.48,3.3 29.61,4.18 29.61,4.43 C24.2 29.83,4.32 v29.84,4.45 | U10.1 20.31,24.14 JP5.4 | v26.67,21.08 25.91,21.84 C10.2 | C2.2 24.02,21.08 | U10.11 16.24,20.81 15.35,19.92 C9.2 | U1.25 U1.24 | U1.45 24.89,11.3 24.27,11.92 C11.2 | U1.15 31.71,22.3 C27.2 31.89,23.23 v31.5,23.62 | C21.2 38.61,23.13 38.61,22.61 v39.24,21.97 | v33.4,11.05 33.4,9.91 33.15,9.65 33.15,8.38 33.31,8.22 U1.65 | 11.83,19.92 11.83,20.81 v11.68,20.95 | v19.56,8.89 20.38,8.06 U9.5 | v15.37,7.75 15.75,7.75 U9.1 | U1.75 38.49,6.22 38.86,6.22 39.5,5.59 v39.5,3.94
  Top 0.305: C9.2 11.83,19.92 | 23.73,13.86 v23.88,13.72 21.73,13.72 C3.2 | 20.73,13.86 INPUT2.2 | C7.2 10.56,20.16 U5.GND | R8.1 13.84,16.64 | 13.84,16.64 v11.68,19.3 | C8.2 15.37,15.11 13.84,16.64 | C6.C 20.07,10.16 | U10.18 22.44,19.5 C2.2 26.42,20.83 v26.67,21.08 26.95,20.8 U1.25 | C12.2 v22.35,18.16
  Top 0.406: OUTPUT2.C 48.26,26.31 | 20.07,10.16 20.07,9.4 v19.56,8.89 | C11.2 24.27,13.32 v23.88,13.72 24,13.84 C26.2 | C23.2 40.64,17.02 v40.89,17.27 | 20.73,13.86 20.85,13.73 C3.2 | INPUT2.2 20.21,13.73 19.94,13.46 U3.2 | U5.GND 10.18,20.3 v10.29,20.95 | 39.75,23.24 39.24,22.73 v39.24,21.97
  Top 0.61: 48.26,26.31 O6.1 | C4.2 C1.2 11.17,10.02 10.56,10.63 | 39.75,23.24 C28.C | C5.C 10.56,10.63 | 10.56,10.63 C7.2 | OUTPUT1.2 INPUT1.2 39.6,4.04 v39.5,3.94
  Top 0.813: C5.C 10.29,10.42 v10.29,9.27
  Bottom 0.61: O6.1 O5.1 O4.1 O3.1 O2.1 O1.1 JP4.1 I1.1
  Bottom 0.813: 48.26,25.4 I1.1 | JP1.4 13.97,2.54 | O7.3 7.62,8
  other vias: 8.89,19.3 8.89,20.95 8.89,22.48 10.29,22.48 11.68,22.48 10.29,19.3
  pour Bottom (isolate 0.305): 6.6,27.94 6.6,0 49.28,0 49.28,27.94
GPS_PPS  (via drill 0.5)
  Top 0.203: U1.67 34.11,6.4 v34.54,5.97 | v24,5.33 24,5.71 22.61,7.11 U9.6
  Route2 0.203: v28.57,4.32 25.02,4.32 v24,5.33
  Route3 0.203: v34.54,5.97 30.23,5.97 v28.57,4.32
GPS_RX  (via drill 0.5)
  Top 0.203: U1.51 26.83,7.4 v26.67,7.24 | U9.3 18.38,5.68 v18.29,5.59 17.65,5.59 15.75,3.68 14.35,3.68 14.1,3.94 14.1,4.32 13.34,5.08 11.43,5.08 O7.2
  Route2 0.203: v18.29,5.59 19.05,4.83 20.45,4.83 21.46,5.84 22.23,5.84 23.37,6.99 26.42,6.99 v26.67,7.24
GPS_TX  (via drill 0.5)
  Top 0.203: U1.52 28.11,9.7 v28.07,9.78 | U9.4 19.38,5.76 v19.56,5.59 18.67,4.7 17.53,4.7 15.88,3.05 14.48,3.05 13.72,3.81 O7.1
  Route2 0.203: v19.56,5.59 20.32,5.59 21.21,6.48 22.1,6.48 23.24,7.62 25.27,7.62 26.42,8.76 27.05,8.76 v28.07,9.78
I1  (via drill 0.5)
  Top 0.203: R22.1 37.97,4.71 v37.21,5.46 | U1.68 34.51,8.67 v34.29,9.02
  Route3 0.203: v34.29,9.02 34.16,9.14 34.16,10.29 34.67,10.79 35.43,10.79 36.58,9.65 36.58,6.86 37.21,6.22 v37.21,5.46
I2  (via drill 0.5)
  Top 0.203: U1.69 34.91,8.37 35.05,8.51 v35.05,10.03 | v36.07,5.84 36.07,5.46 R7.1
  Route3 0.203: v36.07,5.84 36.07,7.49 35.05,8.51 v35.05,10.03
I3
  Top 0.203: U1.70 35.31,5.47 35.94,4.84 R9.1
I4  (via drill 0.5)
  Top 0.203: 34.42,3.41 R10.1 34.67,3.67 v34.67,4.45 | U1.71 35.71,8.79 v35.81,9.02
  Route2 0.203: v35.81,9.02 33.78,6.99 33.78,5.33 v34.67,4.45
I5  (via drill 0.5)
  Top 0.203: U1.79 37.89,10.5 v37.34,10.79 | R11.1 27.56,3.79 v27.56,5.21
  Route2 0.203: v27.56,5.21 27.56,6.1 27.94,6.48 27.94,6.99 33.27,12.32 35.81,12.32 v37.34,10.79
I6  (via drill 0.5)
  Top 0.203: U1.80 38.38,10.9 37.72,11.56 v37.72,11.94 | R12.1 26.29,4.71 v26.29,5.71
  Route2 0.203: v37.72,11.94 36.96,12.7 33.15,12.7 27.56,7.11 27.56,6.99 v26.29,5.71
I7
  Top 0.203: U1.47 26.71,10.5 27.3,9.91 27.3,9.02 25.4,7.11 R13.1
I8
  Top 0.203: U1.48 26.61,10.1 26.92,9.78 26.92,9.14 24.77,6.99 24.77,4.95 24.13,4.32 R14.1
LED1  (via drill 0.5)
  Top 0.203: U1.94 37.86,16.5 v37.72,16.51 | STAT1.C 32.89,23.11 33.78,22.23 v34.42,22.23
  Route2 0.203: v34.42,22.23 37.72,18.92 v37.72,16.51
LED2  (via drill 0.5)
  Top 0.203: U1.98 40.2,18.1 v40.64,18.54 | STAT2.C 36.7,23.11 35.81,22.23 v35.69,22.23
  Route2 0.203: v40.64,18.54 39.37,18.54 v35.69,22.23
MCLR  (via drill 0.5)
  Top 0.203: R15.1 R3.2 C10.1 25.41,24.4 v24.77,23.75
  Route2 0.203: v20.57,15.11 20.57,7.62 19.68,6.73 18.16,6.73 17.27,5.84 17.27,3.81 16,2.54 9.4,2.54 8.13,1.27 JP1.6
  Route3 0.203: v24.77,23.75 20.57,19.56 v20.57,15.11
MPU-CS  (via drill 0.5)
  Top 0.203: R25.1 15.61,24.13 v16.38,24.13 | U1.14 32.11,19.92 32,19.81 29.72,19.81 29.21,19.43 v29.21,17.53
  Route2 0.203: v29.21,17.53 28.45,17.53 26.92,19.05 24.77,19.05 24.13,19.68 24.13,23.11 22.73,24.64 16.76,24.64 v16.38,24.13
MPU-INT  (via drill 0.5)
  Top 0.203: U10.12 16.76,20.14 v16.76,19.43 | U1.66 33.71,8.32 33.53,8.51 33.53,9.53 34.16,10.16 34.16,10.92 34.42,11.18 v34.54,11.56
  Route2 0.203: v16.76,19.43 16.76,18.29 18.29,16.76 25.27,16.76 27.94,14.1 28.57,14.1 v29.46,13.21
  Route3 0.203: v34.54,11.56 32.89,13.21 v29.46,13.21
MPU-MISO  (via drill 0.5)
  Top 0.203: U10.9 14.61,21.84 14.1,21.34 v14.1,20.83 | U1.11 33.31,19.6 32.38,18.67 31.24,18.67 30.48,17.91 30.48,15.75 v29.97,15.24
  Route2 0.203: v29.97,15.24 29.21,14.48 28.07,14.48 25.27,17.27 20.07,17.27 16.64,20.7 14.22,20.7 v14.1,20.83
MPU-MOSI  (via drill 0.5)
  Top 0.203: U10.24 21.33,22.86 v22.35,23.88 | U1.12 32.91,19.7 32.26,19.05 31.11,19.05 30.1,18.03 30.1,16.76 v29.72,16.38
  Route2 0.203: v29.72,16.38 29.08,16.38 27.05,18.41 24.51,18.41 23.37,19.56 23.37,22.86 v22.35,23.88
MPU-SCK  (via drill 0.5)
  Top 0.203: U10.23 22.1,22.35 v22.35,22.61 | U1.10 33.71,19.49 32.51,18.29 31.37,18.29 30.86,17.78 30.86,14.86 30.48,14.48 29.34,14.48 v28.57,15.24
  Route2 0.203: v22.35,22.61 22.35,19.56 24.26,17.65 27.18,17.65 28.57,16.26 v28.57,15.24
N$1
  Top 0.203: STAT1.A 34.16,24.75 R2.1
N$2
  Top 0.203: STAT2.A 35.56,24.75 R4.1
N$3
  Top 0.203: U1.64 32.91,5.7 33.27,5.33 33.27,4.76 Y1.3
N$4
  Top 0.203: JP2.3 40.01,1.27 38.73,2.54 37.7,2.54 R7.2
N$5
  Top 0.203: U10.8 15.38,22.35 R25.2
N$6
  Top 0.203: U1.63 32.51,6.1 32.26,5.84 31.5,5.84 30.99,5.33 30.99,4.76 Y1.1
N$7  (via drill 0.5)
  Top 0.203: U1.13 32.51,19.81 32.13,19.43 30.48,19.43 v29.97,19.05 | R15.2 27.81,22.46 v27.81,22.23
  Route2 0.203: v27.81,22.23 29.97,20.07 v29.97,19.05
N$8
  Top 0.203: JP2.2 37.83,1.27 R9.2
N$9
  Top 0.305: U5.ADJ 12.69,12.42 R1.1 13.11,12.59 R8.2
N$10
  Top 0.203: JP2.1 34.78,1.27 R10.2
N$11
  Top 0.203: JP3.3 31.37,2.92 29.73,2.92 R11.2
N$12
  Top 0.203: R12.2 27.16,2.54 28.57,2.54 29.84,1.27 JP3.2
N$13
  Top 0.203: U10.20 22.45,20.81 C2.1
N$14
  Top 0.203: JP3.1 27.29,1.27 R13.2 | 25.29,3.15 R13.2 | 25.29,3.05 R13.2
N$15  (via drill 0.5)
  other vias: 22.73,4.57
N$16
  Top 0.203: U10.10 15.33,21.31 C9.1
N$17  (via drill 0.5)
  other vias: 14.99,4.57
N$21
  Top 0.203: I1.3 41.4,3.05 38.34,3.05 R22.2
N$35
  Top 0.203: U1.85 40.33,12.9
  Top 0.305: C28.A 41.78,18.54 41.78,13.34 41.34,12.9 40.33,12.9
O1  (via drill 0.5)
  Top 0.203: O1.3 42.04,8.76 36.7,8.76 36.11,8.17 U1.72 | R16.2 39.89,6.53 v39.88,6.54 | v26.1,1.21 25.83,1.21 R14.2
  Route2 0.203: O1.3 42.1,6.54 v39.88,6.54 40.58,5.84 40.58,3.3 39.81,2.54 26.92,2.54 26.1,1.71 v26.1,1.21
O2
  Top 0.203: O2.3 41.68,9.3 U1.76
O3
  Top 0.203: O3.3 41.4,12.19 41.4,10.54 40.56,9.7 U1.77
O4  (via drill 0.5)
  Top 0.203: U1.78 38.29,10.1 v37.72,9.65
  Route3 0.203: O4.3 44.45,15.88 44.45,10.16 43.56,9.27 38.1,9.27 v37.72,9.65
O5  (via drill 0.5)
  Top 0.203: U1.81 40.27,11.3 v40.64,10.92
  Route3 0.203: v40.64,10.92 40.89,10.92 42.04,12.06 42.04,19.18 O5.3
O6  (via drill 0.5)
  Top 0.203: U1.82 40.27,11.7 v40.64,12.06
  Route3 0.203: v40.64,12.06 41.66,13.08 41.66,21.97 O6.3
PGEC2  (via drill 0.5)
  Top 0.203: U1.74 36.91,8.21 37.08,8.38 37.85,8.38 v38.35,7.87
  Route2 0.203: JP1.2 18.41,1.27 20.13,2.98 37.4,2.98 39.37,4.95 39.37,5.78 38.35,6.79 v38.35,7.87
PGED2  (via drill 0.5)
  Top 0.203: v38.48,5.46 37.72,6.35 36.7,6.35 36.51,6.54 U1.73
  Route2 0.203: JP1.3 17.4,3.43 36.83,3.43 38.48,5.08 v38.48,5.46
RG1  (via drill 0.5)
  Top 0.203: U1.89 37.57,14.5 v36.83,15.24 | v39.88,7.81 39.89,7.83 R16.1
  Route2 0.203: v36.83,15.24 39.88,12.19 v39.88,7.81
RX2  (via drill 0.5)
  Top 0.203: U1.49 24.47,9.7 23.75,10.41 v22.48,10.41
  Route2 0.203: JP5.2 11.05,25.02 9.14,25.02 8,23.88 8,17.78 9.91,15.88 9.91,11.81 9.4,11.3 9.4,7.11 JP6.2 11.43,7.62 12.95,7.62 14.22,8.89 v14.86,8.89
  Route3 0.203: v22.48,10.41 16.38,10.41 v14.86,8.89
SCK1  (via drill 0.5)
  Top 0.203: U1.55 29.31,8.74 30.73,10.16 v30.73,11.43
  Route2 0.203: v33.15,17.4 33.15,13.97 30.73,11.56 v30.73,11.43
  Bottom 0.203: JP8.1 39.37,24.13 35.05,24.13 32.77,21.84 32.77,18.41 33.15,18.03 v33.15,17.4
SCL2  (via drill 0.5)
  Top 0.203: R5.1 14.86,16.88 14.86,16.76 15.75,15.88 v16,15.88 | U1.58 30.51,8.41 v31.37,9.27
  Route2 0.203: v27.3,12.45 23.75,12.45 21.59,14.61 21.59,15.24 20.95,16 20.19,16 20.07,15.88 v16,15.88
  Route3 0.203: v31.37,9.27 31.37,10.79 31.62,11.05 31.62,11.81 31.11,12.32 30.35,12.32 29.97,11.94 28.83,11.94 28.32,12.45 v27.3,12.45
  Bottom 0.203: v16,15.88 15.62,16.26 13.72,16.26 TP-SCL2.P$1
SDA2  (via drill 0.5)
  Top 0.203: R6.1 15.99,16.89 v17.02,16.89 | U1.59 30.91,8.31 30.99,8.38 31.88,8.38 32.38,8.89 v32.38,10.29
  Route2 0.203: v28.19,13.34 25.65,13.34 23.88,15.11 22.48,15.11 21.21,16.38 17.53,16.38 v17.02,16.89
  Route3 0.203: v28.19,13.34 28.19,13.21 29.08,12.32 29.84,12.32 30.35,12.83 31.62,12.83 32.38,12.06 v32.38,10.29
  Bottom 0.203: v17.02,16.89 17.02,15.24 16.64,14.86 15.75,14.86 14.99,15.62 TP-SDA2.P$1
SDI1  (via drill 0.5)
  Top 0.203: U1.54 28.91,8.85 29.34,9.27 29.34,10.03 v29.84,10.54
  Route2 0.203: v29.84,10.54 29.84,11.81 31.62,13.59 v31.62,17.4
  Bottom 0.203: JP8.3 36.58,26.67 32,22.1 32,18.41 31.62,18.03 v31.62,17.4
SDO1  (via drill 0.5)
  Top 0.203: U1.53 28.51,8.95 28.96,9.4 28.96,10.92 32.38,14.35 v32.38,16.51
  Bottom 0.203: JP8.2 39.37,24.64 39.24,24.51 34.92,24.51 32.38,21.97 v32.38,16.51
SS1  (via drill 0.5)
  Top 0.203: U1.23 28.51,19.37 v28.45,19.3
  Bottom 0.203: JP8.4 32.38,26.67 30.35,24.64 29.84,24.64 28.7,23.5 28.7,19.56 v28.45,19.3
SVCC  (via drill 0.5)
  Top 0.61: OUTPUT2.A 45.23,23.98 O6.2 | O1.2 45.72,7.52 | OUTPUT1.1 41.96,5.3 v43.81,5.3
  Top 0.813: O6.2 O5.2 O4.2 O3.2 O2.2 O1.2
  Route3 0.813: v43.81,5.3 45.72,7.21 O1.2
  Bottom 0.61: SJ1.2 42.9,5.21 42.93,5.21 43.02,5.3 v43.81,5.3
  Bottom 0.813: 45.72,7.27 O1.2
TX2  (via drill 0.5)
  Top 0.203: U1.50 23.6,9.3 v22.99,9.27
  Route2 0.203: JP5.1 9.65,26.67 7.62,24.64 7.62,8.26 8.89,6.99 8.89,5.71 9.53,5.08 11.43,5.08 JP6.1 16.64,6.35 18.16,7.87 v18.16,8.89
  Route3 0.203: v22.99,9.27 20.32,9.27 19.94,9.65 18.92,9.65 v18.16,8.89
VCC  (via drill 0.5)
  Top 0.203: U3.1 19.41,12.43
  Top 0.305: v22.35,8.13 21.59,8.89 21.59,12.3 C3.1 | U3.1 18.35,12.51 18.03,12.83 18.03,14.1 17.72,14.41 U3.4
  Top 0.406: C3.1 INPUT2.1 19.33,12.43 U3.1
  Top 0.61: JP4.2 I1.2 | C7.1 8.64,12.19 | INPUT1.1 v43.82,4.04
  Top 0.813: 9.24,13.97 U5.VIN U5.EN 8.6,14 8.64,13.97 8.64,12.19 8.64,11.51 C5.A | 7.87,10.23 C5.A | v8.51,9.02 7.62,9.91 C5.A
  Route3 0.305: v22.35,8.13 27.69,2.79
  Route3 0.813: v8.51,9.02 9.4,8.13 13.46,8.13 18.8,2.79 27.69,2.79 42.58,2.79 v43.82,4.04 45.31,4.04 JP4.2
  Bottom 0.61: SJ1.1 v43.82,4.04

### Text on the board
tPlace: GPS
bPlace: TX2 | RX2 | 3.3V | GND | AN18 | AN17 | AN16 | AN15 | SS | SDI | SDO | SCK | ~ | + | - | OUT6 | OUT5 | SCL2 | UDB5mini | OUT4 | v1.0 | SDA2 | OUT3 | 3.3V | GND | Octopilot / Electronics / LLC | OUT2 | - | RX2 | TX2 | - | GRX | GTX | OUT1 | SVCC / VCC | PROG | 5V | IN7 | IN6 | IN5 | IN4 | IN3 | IN2 | IN1 | + | -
